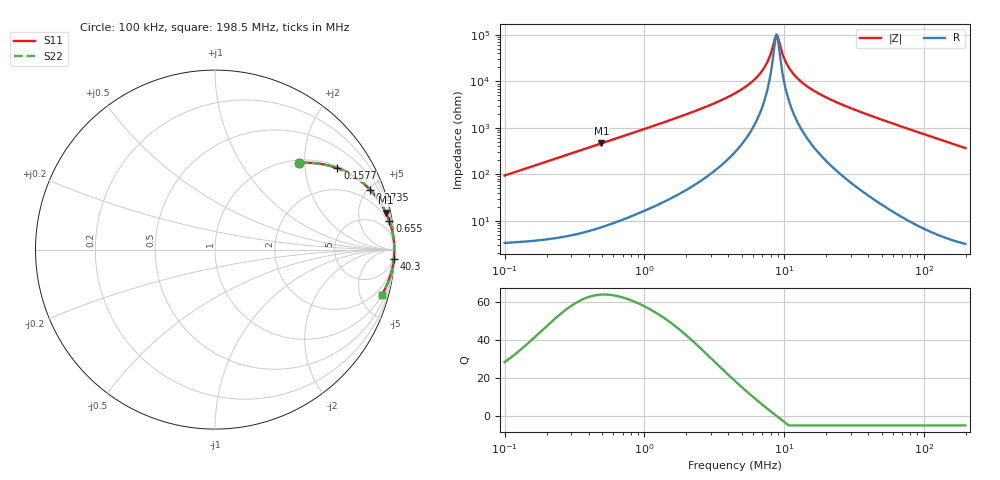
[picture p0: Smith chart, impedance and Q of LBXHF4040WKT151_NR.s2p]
! LBXHF4040WKT151_NR  S-PARAMETER MODEL  ( Standard Model )
! Model Generated by TAIYO YUDEN Corporation (http://www.ty-top.com)
! Version 1.0
! TAIYO YUDEN Control No. 20221109
! Copyright(c) 2022 TAIYO YUDEN CO.,LTD. All Rights Reserved.
! Product Description (link to TY-COMPAS)
! https://ds.yuden.co.jp/TYCOMPAS/or/detail?pn=LBXHF4040WKT151MNR&u=M
! Products Name : Inductors
! Characteristics :
!  Inductance : 150 [uH] , SRF(min) : 7.0 [MHz] , DC Resistance(max) : 2.364 [Ohm]
!  Rated Current : Saturation  390 [mA] , Temp Rise  250 [mA]
!  Case Size : 4.0 x 4.0 / 0.157 x 0.157 [mm/inch] , Thickness : 2.0 / 0.079 [mm/inch]
!  (Conditions: Temperature = 25 [degC] , DC Bias Current = 0 [A])
! External Node Assignments :
!  1  o---GGG---o  2
! GND o---------o GND
! Frequency Range : 0.1MHz  -  198.534594MHz  [ 402 STEP ]
# MHz S RI R 50
! Freq[MHz].  S11 Real  S11 Imag  S21 Real  S21 Imag  S12 Real  S12 Imag  S22 Real  S22 Imag
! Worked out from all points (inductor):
!   401 points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, 100 kHz to 198.5 MHz, reference 50 ohm
!   read as one part in series: L = 149 uH near 103.9 kHz
!   highest Q = 64 at 492.7 kHz (marker M1), where L = 149 uH
!   self-resonance near 8.825 MHz
!   S11 on the Smith chart (normalised r, x): 100 kHz: 1.07, +1.88; 157.7 kHz: 1.07, +2.96; 273.5 kHz: 1.09, +5.13; 655 kHz: 1, +12; 40.3 MHz: 2, -38; 198.5 MHz: 1.06, -7.33
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0.1  0.4707 0.4818  0.5293 -0.4818  0.5293 -0.4818  0.4707 0.4818
0.157714  0.6823 0.4533  0.3177 -0.4533  0.3177 -0.4533  0.6823 0.4533
0.273504  0.8635 0.3345  0.1365 -0.3345  0.1365 -0.3345  0.8635 0.3345
0.356769  0.9142 0.2721  0.0858 -0.2721  0.0858 -0.2721  0.9142 0.2721
0.492658  0.9523 0.2055  0.0477 -0.2055  0.0477 -0.2055  0.9523 0.2055
0.65496  0.9718 0.1577  0.0282 -0.1577  0.0282 -0.1577  0.9718 0.1577
1.272844  0.9917 0.0819  0.00831 -0.0819  0.00831 -0.0819  0.9917 0.0819
2.772065  0.9977 0.0349  0.00229 -0.0349  0.00229 -0.0349  0.9977 0.0349
4.541117  0.9987 0.0174  0.00128 -0.0174  0.00128 -0.0174  0.9987 0.0174
5.812224  0.9989 0.0105  0.00108 -0.0105  0.00108 -0.0105  0.9989 0.0105
6.895149  0.999 0.0061  0.001 -0.0061  0.001 -0.0061  0.999 0.0061
7.727005  0.999 0.00328  0.000981 -0.00328  0.000981 -0.00328  0.999 0.00328
8.496385  0.999 0.000967  0.000974 -0.000967  0.000974 -0.000967  0.999 0.000967
8.825176  0.999 4.53e-05  0.000975 -4.53e-05  0.000975 -4.53e-05  0.999 4.53e-05
9.16669  0.999 -0.000876  0.000977 0.000876  0.000977 0.000876  0.999 -0.000876
10.07942  0.999 -0.00319  0.000989 0.00319  0.000989 0.00319  0.999 -0.00319
11.08303  0.999 -0.00552  0.00101 0.00552  0.00101 0.00552  0.999 -0.00552
12.90076  0.9989 -0.00937  0.00106 0.00937  0.00106 0.00937  0.9989 -0.00937
15.89665  0.9988 -0.015  0.00119 0.015  0.00119 0.015  0.9988 -0.015
40.29866  0.9963 -0.0526  0.00373 0.0526  0.00373 0.0526  0.9963 -0.0526
56.71438  0.9932 -0.0756  0.00677 0.0756  0.00677 0.0756  0.9932 -0.0756
198.5346  0.9288 -0.2529  0.0712 0.2529  0.0712 0.2529  0.9288 -0.2529
